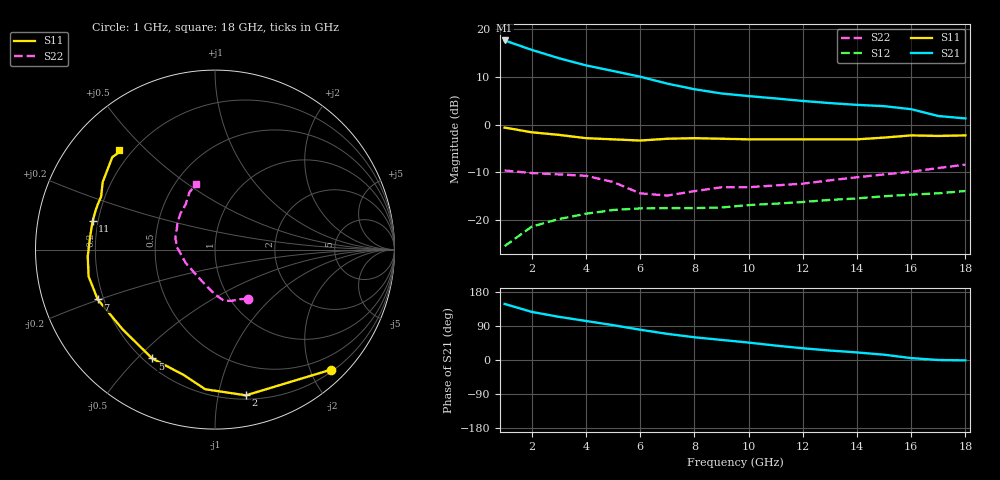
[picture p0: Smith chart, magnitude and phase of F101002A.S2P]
!ATF-10100
!S-PARAMETERS at Vds=2V  Id=25mA.  LAST UPDATED 07-22-92
# ghz s ma r 50
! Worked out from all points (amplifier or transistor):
!   18 points, 1 GHz to 18 GHz, reference 50 ohm
!   highest |S21| = 17.7 dB at 1 GHz (marker M1)
!   |S21| within 3 dB of that: start of sweep to 2.587 GHz
!   unconditionally stable (mu >= 1): 11.5 GHz to 14.7 GHz; 16.74 GHz to end of sweep
!   at 4 GHz: K = 0.52, MSG = 15.6 dB, |S12| = -18.7 dB
!   at 10 GHz: K = 0.97, MSG = 11.4 dB, |S12| = -16.9 dB
!   at 18 GHz: K = 1.02, MAG = 6.7 dB, |S12| = -13.9 dB
!   lowest NFmin = 0.30 dB at 100 MHz
!   S11 on the Smith chart (normalised r, x): 1 GHz: 0.24, -2.34; 2 GHz: 0.23, -1.21; 5 GHz: 0.23, -0.55; 7 GHz: 0.18, -0.20; 11 GHz: 0.18, +0.11; 18 GHz: 0.15, +0.42
1  0.93 -46.0  7.63 148.0  0.053 64.0  0.33 -56.0
2  0.83 -78.0  6.08 127.0  0.085 52.0  0.31 -63.0
3  0.78 -94.0  4.97 114.0  0.102 45.0  0.3 -72.0
4  0.72 -104.0  4.18 103.0  0.116 41.0  0.29 -80.0
5  0.7 -120.0  3.65 92.0  0.127 36.0  0.25 -90.0
6  0.68 -139.0  3.18 80.0  0.132 31.0  0.19 -113.0
7  0.71 -157.0  2.69 69.0  0.133 25.0  0.18 -156.0
8  0.72 -168.0  2.35 60.0  0.133 22.0  0.2 -178.0
9  0.71 -177.0  2.12 53.0  0.135 19.0  0.22 174.0
10  0.7 175.0  1.99 46.0  0.143 17.0  0.22 169.0
11  0.7 167.0  1.88 38.0  0.148 15.0  0.23 164.0
12  0.7 162.0  1.77 31.0  0.154 13.0  0.24 153.0
13  0.7 159.0  1.68 25.0  0.162 11.0  0.26 143.0
14  0.7 155.0  1.61 20.0  0.168 10.0  0.28 133.0
15  0.73 149.0  1.56 14.0  0.177 8.0  0.3 123.0
16  0.77 138.0  1.45 5.0  0.184 6.0  0.32 119.0
17  0.76 134.0  1.23 0.0  0.19 5.0  0.35 114.0
18  0.77 134.0  1.16 -1.0  0.201 4.0  0.38 106.0
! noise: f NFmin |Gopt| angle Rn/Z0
0.1  0.3  0.99  1  0.5
2  0.4  0.55  27  0.29
4  0.55  0.39  65  0.22
6  0.8  0.41  105  0.16
8  1  0.46  144  0.1
12  1.3  0.5  174  0.09
